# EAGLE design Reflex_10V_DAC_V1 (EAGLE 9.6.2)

## Sheet 1 of 3: Analog Circuits
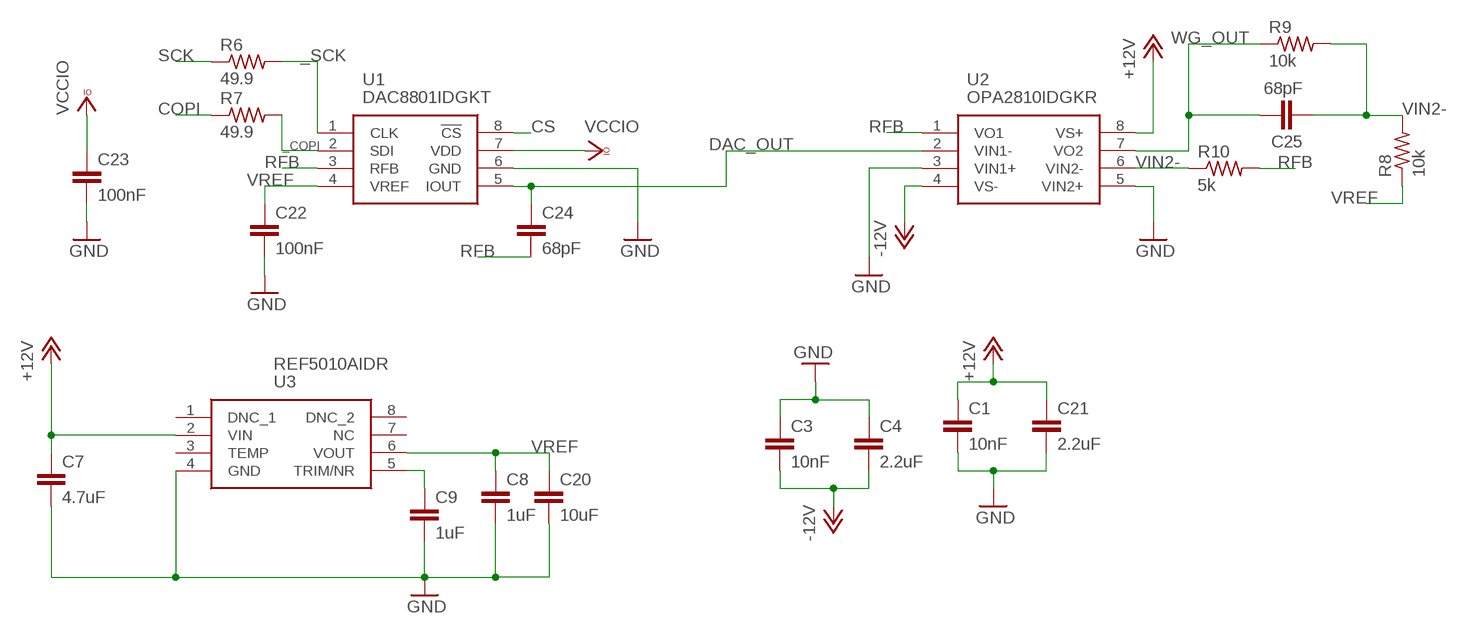
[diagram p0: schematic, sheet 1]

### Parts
C1  10nF  C-EUC0603  [C0603]
C3  10nF  C-EUC0603  [C0603]
C4  2.2uF  C-EUC0603  [C0603]
C7  4.7uF  C-EUC0603  [C0603]
C8  1uF  C-EUC0603  [C0603]
C9  1uF  C-EUC0603  [C0603]
C20  10uF  C-EUC0603  [C0603]
C21  2.2uF  C-EUC0603  [C0603]
C22  100nF  C-EUC0603  [C0603]
C23  100nF  C-EUC0603  [C0603]
C24  68pF  C-EUC0603  [C0603]
C25  68pF  C-EUC0603  [C0603]
R6  49.9  R-US_R0603  [R0603]
R7  49.9  R-US_R0603  [R0603]
R8  10k  R-US_R0603  [R0603]
R9  10k  R-US_R0603  [R0603]
R10  5k  R-US_R0603  [R0603]
U1  DAC8801IDGKT  [SOP65P490X110-8N]
U2  OPA2810IDGKR  [SOP65P490X110-8N]
U3  REF5010AIDR  [SOIC127P600X175-8N]

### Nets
+12V: C1.1 C7.1 C21.1 U2.8(VS+) U3.2(VIN) ; also sheet 2
-12V: C3.2 C4.2 U2.4(VS-) ; also sheet 2
_COPI: R7.2 U1.2(SDI)
_SCK: R6.2 U1.1(CLK)
COPI: R7.1 ; also sheet 3
CS: U1.8(!CS) ; also sheet 3
DAC_OUT: C24.1 U1.5(IOUT) U2.2(VIN1-)
GND: C1.2 C3.1 C4.1 C7.2 C8.2 C9.2 C20.2 C21.2 C22.2 C23.2 U1.6(GND) U2.3(VIN1+) U2.5(VIN2+) U3.4(GND) ; also sheet 2,3
N$8: C9.1 U3.5(TRIM/NR)
RFB: C24.2 R10.2 U1.3(RFB) U2.1(VO1)
SCK: R6.1 ; also sheet 3
VCCIO: C23.1 U1.7(VDD) ; also sheet 3
VIN2-: C25.2 R8.2 R9.2 R10.1 U2.6(VIN2-)
VREF: C8.1 C20.1 C22.1 R8.1 U1.4(VREF) U3.6(VOUT) ; also sheet 3
WG_OUT: C25.1 R9.1 U2.7(VO2) ; also sheet 3
Unconnected: U3.1(DNC_1) U3.3(TEMP) U3.7(NC) U3.8(DNC_2)

## Sheet 2 of 3: Power Circuits
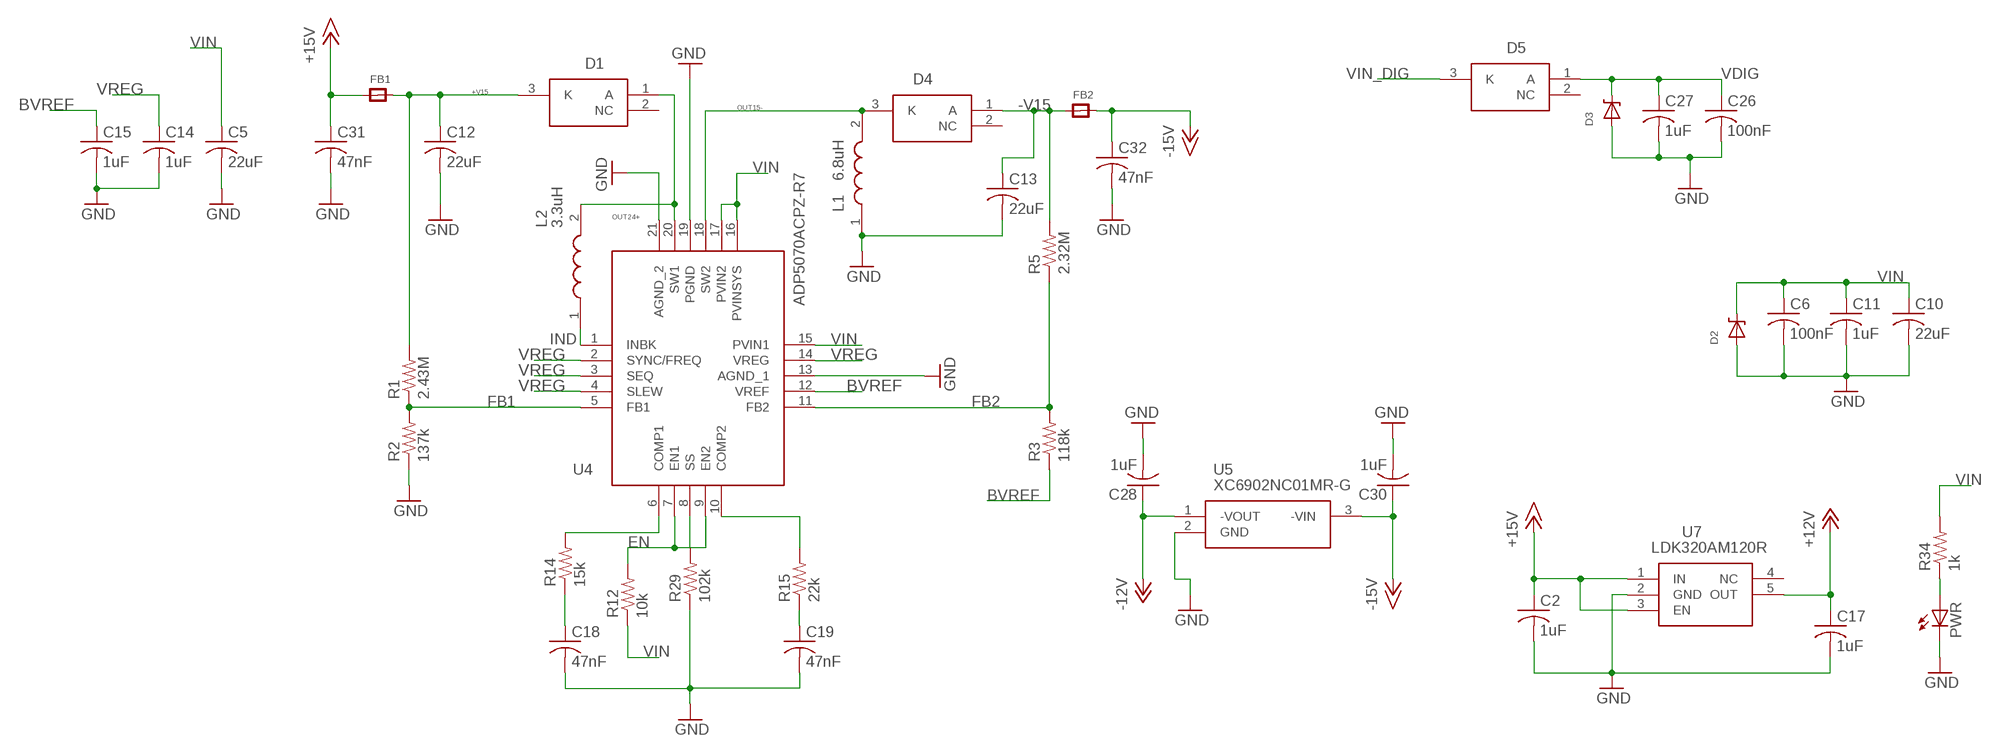
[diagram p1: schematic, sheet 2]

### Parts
C2  1uF  C-USC0603  [C0603]
C5  22uF  C-USC0603  [C0603]
C6  100nF  C-USC0603  [C0603]
C10  22uF  C-USC0603  [C0603]
C11  1uF  C-USC0603  [C0603]
C12  22uF  C-USC0805  [C0805]
C13  22uF  C-USC0805  [C0805]
C14  1uF  C-USC0603  [C0603]
C15  1uF  C-USC0603  [C0603]
C17  1uF  C-USC0603  [C0603]
C18  47nF  C-USC0603  [C0603]
C19  47nF  C-USC0603  [C0603]
C26  100nF  C-USC0603  [C0603]
C27  1uF  C-USC0603  [C0603]
C28  1uF  C-USC0603  [C0603]
C30  1uF  C-USC0603  [C0603]
C31  47nF  C-USC0603  [C0603]
C32  47nF  C-USC0603  [C0603]
D1  BAT54WFILMY  [SOT65P210X110-3N]
D2  DDZ5V6ASF  [DDZ5V6ASF]
D3  DDZ5V6ASF  [DDZ5V6ASF]
D4  BAT54WFILMY  [SOT65P210X110-3N]
D5  BAT54WFILMY  [SOT65P210X110-3N]
FB1  FERRITE  [0603]
FB2  FERRITE  [0603]
L1  6.8uH  MLZ2012M6R8HTD25  [INDC2012X105N]
L2  3.3uH  MLZ2012M4R7HT000  [INDC2012X145N]
PWR  LEDCHIPLED_0603  [CHIPLED_0603]
R1  2.43M  R-US_R0603  [R0603]
R2  137k  R-US_R0603  [R0603]
R3  118k  R-US_R0603  [R0603]
R5  2.32M  R-US_R0603  [R0603]
R12  10k  R-US_R0603  [R0603]
R14  15k  R-US_R0603  [R0603]
R15  22k  R-US_R0603  [R0603]
R29  102k  R-US_R0603  [R0603]
R34  1k  R-US_R0603  [R0603]
U4  ADP5070ACPZ-R7  [QFN50P400X400X80-21N]
U5  XC6902NC01MR-G  [SOT95P280X130-3N]
U7  LDK320AM120R  [SOT95P280X145-5N]

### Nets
+12V: C17.1 U7.5(OUT) ; also sheet 1
+15V: C2.1 C31.1 FB1.1 U7.1(IN) U7.3(EN)
+V15: C12.1 D1.3(K) FB1.2 R1.2
-12V: C28.1 U5.1(-VOUT) ; also sheet 1
-15V: C30.1 C32.1 FB2.2 U5.3(-VIN)
-V15: C13.1 D4.1(A) FB2.1 R5.2
BVREF: C15.1 R3.1 U4.12(VREF)
EN: R12.2 U4.7(EN1) U4.9(EN2) ; also sheet 3
FB1: R1.1 R2.2 U4.5(FB1)
FB2: R3.2 R5.1 U4.11(FB2)
GND: C2.2 C5.2 C6.2 C10.2 C11.2 C12.2 C13.2 C14.2 C15.2 C17.2 C18.2 C19.2 C26.2 C27.2 C28.2 C30.2 C31.2 C32.2 D2.P$1(A) D3.P$1(A) L1.1 PWR.C R2.1 R29.1 U4.13(AGND_1) U4.19(PGND) U4.21(AGND_2) U5.2(GND) U7.2(GND) ; also sheet 1,3
IND: L2.1 U4.1(INBK)
N$19: PWR.A R34.1
N$20: R29.2 U4.8(SS)
N$29: C18.1 R14.1
N$30: R14.2 U4.6(COMP1)
N$31: C19.1 R15.1
N$32: R15.2 U4.10(COMP2)
OUT15-: D4.3(K) L1.2 U4.18(SW2)
OUT24+: D1.1(A) L2.2 U4.20(SW1)
VDIG: C26.1 C27.1 D3.P$2(C) D5.1(A) ; also sheet 3
VIN: C5.1 C6.1 C10.1 C11.1 D2.P$2(C) R12.1 R34.2 U4.15(PVIN1) U4.16(PVINSYS) U4.17(PVIN2) ; also sheet 3
VIN_DIG: D5.3(K) ; also sheet 3
VREG: C14.1 U4.2(SYNC/FREQ) U4.3(SEQ) U4.4(SLEW) U4.14(VREG)
Unconnected: D1.2(NC) D4.2(NC) D5.2(NC) U7.4(NC)

## Sheet 3 of 3: Connectors and analog switch
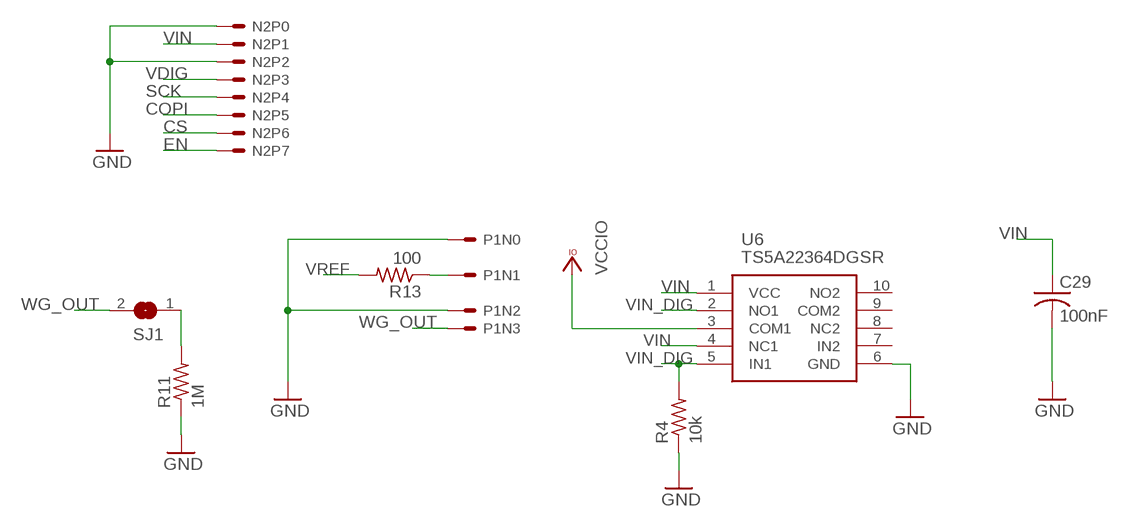
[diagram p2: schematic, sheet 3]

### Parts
C29  100nF  C-USC0603  [C0603]
N2  8PINHEADER  [8PINHEADER]
P1  4PINHEADER  [4PINHEADER]
R4  10k  R-US_R0603  [R0603]
R11  1M  R-US_R0603  [R0603]
R13  100  R-US_R0603  [R0603]
SJ1  SOLDERJUMPER  [SOLDERJUMPER_ARROW_NOPASTE]
U6  TS5A22364DGSR  [SOP50P490X110-10N]

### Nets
COPI: N2.P5 ; also sheet 1
CS: N2.P6 ; also sheet 1
EN: N2.P7 ; also sheet 2
GND: C29.2 N2.P0 N2.P2 P1.N0 P1.N2 R4.1 R11.1 U6.6(GND) ; also sheet 1,2
N$1: R11.2 SJ1.1
N$2: P1.N1 R13.1
SCK: N2.P4 ; also sheet 1
VCCIO: U6.3(COM1) ; also sheet 1
VDIG: N2.P3 ; also sheet 2
VIN: C29.1 N2.P1 U6.1(VCC) U6.4(NC1) ; also sheet 2
VIN_DIG: R4.2 U6.2(NO1) U6.5(IN1) ; also sheet 2
VREF: R13.2 ; also sheet 1
WG_OUT: P1.N3 SJ1.2 ; also sheet 1
Unconnected: U6.7(IN2) U6.8(NC2) U6.9(COM2) U6.10(NO2)

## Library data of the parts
C1 C3 C4 C7-C9 C20-C25 = rcl:C-EU: CAPACITOR, European symbol; SPICEPREFIX: C
C2 C5 C6 C10-C15 C17-C19 C26-C32 = rcl:C-US: CAPACITOR, American symbol; SPICEPREFIX: C
D1 D4 D5 = SamacSys_Parts:BAT54WFILMY: Automotive 40 V, 300 mA General purpose Small Signal Schottky Diode Source: Datasheet; DESCRIPTION: Automotive 40 V, 300 mA General purpose Small Signal Schottky Diode; HEIGHT: 1.1mm; MANUFACTURER_NAME: STMicroelectronics; MANUFACTURER_PART_NUMBER: BAT54WFILMY; MOUSER_PART_NUMBER: 511-BAT54WFILMY; MOUSER_PRICE-STOCK: https://www.mouser.co.uk/ProductDetail/STMicroelectronics/BAT54WFILMY?qs=aA7MvVR8Lz8Zb51n0tQT7w%3D%3D
D2 D3 = ForceTronics:DDZ5V6ASF: DDZ5V6ASF 5.42 Zener Diode
FB1 FB2 = microbuilder:FERRITE: Ferrite Bead
L1 = SamacSys_Parts:MLZ2012M6R8HTD25: The MLZ series include inductors for decoupling circuits that have top-class DC superimposition characteristics and low DC resistance. They are compatible with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; DESCRIPTION: The MLZ series include inductors for decoupling circuits that have top-class DC superimposition characteristics and low DC resistance. They are compatible with wide frequency band noise, from low to high frequency. H type products have a rated current that is equivalent to that of wound coils. W type products are the new standard type products that have both large current and low resistance. L type products have a resistance up to 60% lower than W type products. Operating temperature range: 55 to +125; HEIGHT: 1.05mm; MANUFACTURER_NAME: TDK; MANUFACTURER_PART_NUMBER: MLZ2012M6R8HTD25; MOUSER_PART_NUMBER: 810-MLZ2012M6R8HTD25; MOUSER_PRICE-STOCK: https://www.mouser.co.uk/ProductDetail/TDK/MLZ2012M6R8HTD25?qs=YdQ7Kj7W0bzS66dbWGL5AA%3D%3D
L2 = SamacSys_Parts:MLZ2012M4R7HT000: Inductor Power Shielded Multi-Layer 4.7uH 20% 2MHz Ferrite 0.4A 0.442Ohm DCR 0805 T/R; DESCRIPTION: Inductor Power Shielded Multi-Layer 4.7uH 20% 2MHz Ferrite 0.4A 0.442Ohm DCR 0805 T/R; HEIGHT: 1.45mm; MANUFACTURER_NAME: TDK; MANUFACTURER_PART_NUMBER: MLZ2012M4R7HT000; MOUSER_PART_NUMBER: 810-MLZ2012M4R7HT000; MOUSER_PRICE-STOCK: https://www.mouser.co.uk/ProductDetail/TDK/MLZ2012M4R7HT000?qs=%2FPzWLGNeQ%252BgQgMrI9kQ17A%3D%3D
N2 = ForceTronics:8PINHEADER: 8 pin header with 2.54mm spacing
P1 = ForceTronics:4PINHEADER
PWR = adafruit:LED: LED
R1-R15 R29 R34 = rcl:R-US_: RESISTOR, American symbol; SPICEPREFIX: R
SJ1 = microbuilder:SOLDERJUMPER: SMD Solder JUMPER; BOM: EXCLUDE
U1 = SamacSys_Parts:DAC8801IDGKT: 14-Bit, Single Channel, Serial Interface, Multiplying Digital-to-Analog Converter Source: Datasheet; DESCRIPTION: 14-Bit, Single Channel, Serial Interface, Multiplying Digital-to-Analog Converter; HEIGHT: 1.1mm; MANUFACTURER_NAME: Texas Instruments; MANUFACTURER_PART_NUMBER: DAC8801IDGKT; MOUSER_PART_NUMBER: 595-DAC8801IDGKT; MOUSER_PRICE-STOCK: https://www.mouser.co.uk/ProductDetail/Texas-Instruments/DAC8801IDGKT?qs=vul0MlC%2Fa1fY4dNbzQeDsA%3D%3D
U2 = SamacSys_Parts:OPA2810IDGKR: High Performance Low Cost Rail-to-Rail Input/Output HV FET Op Amps Source: Datasheet; DESCRIPTION: High Performance Low Cost Rail-to-Rail Input/Output HV FET Op Amps; HEIGHT: 1.1mm; MANUFACTURER_NAME: Texas Instruments; MANUFACTURER_PART_NUMBER: OPA2810IDGKR; MOUSER_PART_NUMBER: 595-OPA2810IDGKR; MOUSER_PRICE-STOCK: https://www.mouser.co.uk/ProductDetail/Texas-Instruments/OPA2810IDGKR?qs=YCa%2FAAYMW02J4dMmTpJlwg%3D%3D
U3 = SamacSys_Parts:REF5010AIDR: Low Noise, Very Low Drift, Precision Series Voltage Reference Source: Datasheet; DESCRIPTION: Low Noise, Very Low Drift, Precision Series Voltage Reference; HEIGHT: 1.75mm; MANUFACTURER_NAME: Texas Instruments; MANUFACTURER_PART_NUMBER: REF5010AIDR; MOUSER_PART_NUMBER: 595-REF5010AIDR; MOUSER_PRICE-STOCK: https://www.mouser.co.uk/ProductDetail/Texas-Instruments/REF5010AIDR?qs=XGzIaZb%2FFYJH5K17rhHGBw%3D%3D
U4 = SamacSys_Parts:ADP5070ACPZ-R7: ANALOG DEVICES - ADP5070ACPZ-R7 - DC/DC CONV, BOOST/INVERTING, LFCSP-20 Source: Datasheet; DESCRIPTION: ANALOG DEVICES - ADP5070ACPZ-R7 - DC/DC CONV, BOOST/INVERTING, LFCSP-20; HEIGHT: 0.8mm; MANUFACTURER_NAME: Analog Devices; MANUFACTURER_PART_NUMBER: ADP5070ACPZ-R7; MOUSER_PART_NUMBER: 584-ADP5070ACPZ-R7; MOUSER_PRICE-STOCK: https://www.mouser.co.uk/ProductDetail/Analog-Devices/ADP5070ACPZ-R7?qs=Ky1INM14uHq5PX2hKR%252Babw%3D%3D
U5 = SamacSys_Parts:XC6902NC01MR-G: Maximum Output Current : 200mA Input Voltage Range : -2.4 ~ -16V Output Voltage Range : -0.9 ~ -12V Accuracy : +/-1.5% for -2.0V ~ -12V +/-30mV (-0.9V ~ -1.95V) Temperature Stability : TYP. +/-50ppm/ Dropout Voltage : 400mVIOUT=100mA Low Power Consumption : 100uA Protection Circuits : Current Limit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; DESCRIPTION: Maximum Output Current : 200mA Input Voltage Range : -2.4 ~ -16V Output Voltage Range : -0.9 ~ -12V Accuracy : +/-1.5% for -2.0V ~ -12V +/-30mV (-0.9V ~ -1.95V) Temperature Stability : TYP. +/-50ppm/ Dropout Voltage : 400mVIOUT=100mA Low Power Consumption : 100uA Protection Circuits : Current Limit 350mA TYP. Foldback Thermal Shutdown (150) Output Capacitor : Ceramic Capacitor Compatible Operating Ambient Temperature : -40 ~ 85 Packages : SOT-23, SOT-89, USP-6C Environmentally Friendly : EU Ro; HEIGHT: 1.3mm; MANUFACTURER_NAME: Torex; MANUFACTURER_PART_NUMBER: XC6902NC01MR-G
U6 = SamacSys_Parts:TS5A22364DGSR: Analog Switch ICs 0.65-Ohm Dual SPDT Analog Switch Source: Datasheet; DESCRIPTION: Analog Switch ICs 0.65-Ohm Dual SPDT Analog Switch; HEIGHT: 1.1mm; MANUFACTURER_NAME: Texas Instruments; MANUFACTURER_PART_NUMBER: TS5A22364DGSR; MOUSER_PART_NUMBER: 595-TS5A22364DGSR; MOUSER_PRICE-STOCK: https://www.mouser.co.uk/ProductDetail/Texas-Instruments/TS5A22364DGSR?qs=9F2IyUQaA%2FhbjQmUI4VB%2FQ%3D%3D
U7 = SamacSys_Parts:LDK320AM120R: STMICROELECTRONICS - LDK320AM120R - LDO, FIXED, 12V, 0.2A, SOT-23-5 Source: Datasheet; DESCRIPTION: STMICROELECTRONICS - LDK320AM120R - LDO, FIXED, 12V, 0.2A, SOT-23-5; HEIGHT: 1.45mm; MANUFACTURER_NAME: STMicroelectronics; MANUFACTURER_PART_NUMBER: LDK320AM120R; MOUSER_PART_NUMBER: 511-LDK320AM120R; MOUSER_PRICE-STOCK: https://www.mouser.co.uk/ProductDetail/STMicroelectronics/LDK320AM120R?qs=wd5RIQLrsJgIHDY%252B%2Fbe1dQ%3D%3D

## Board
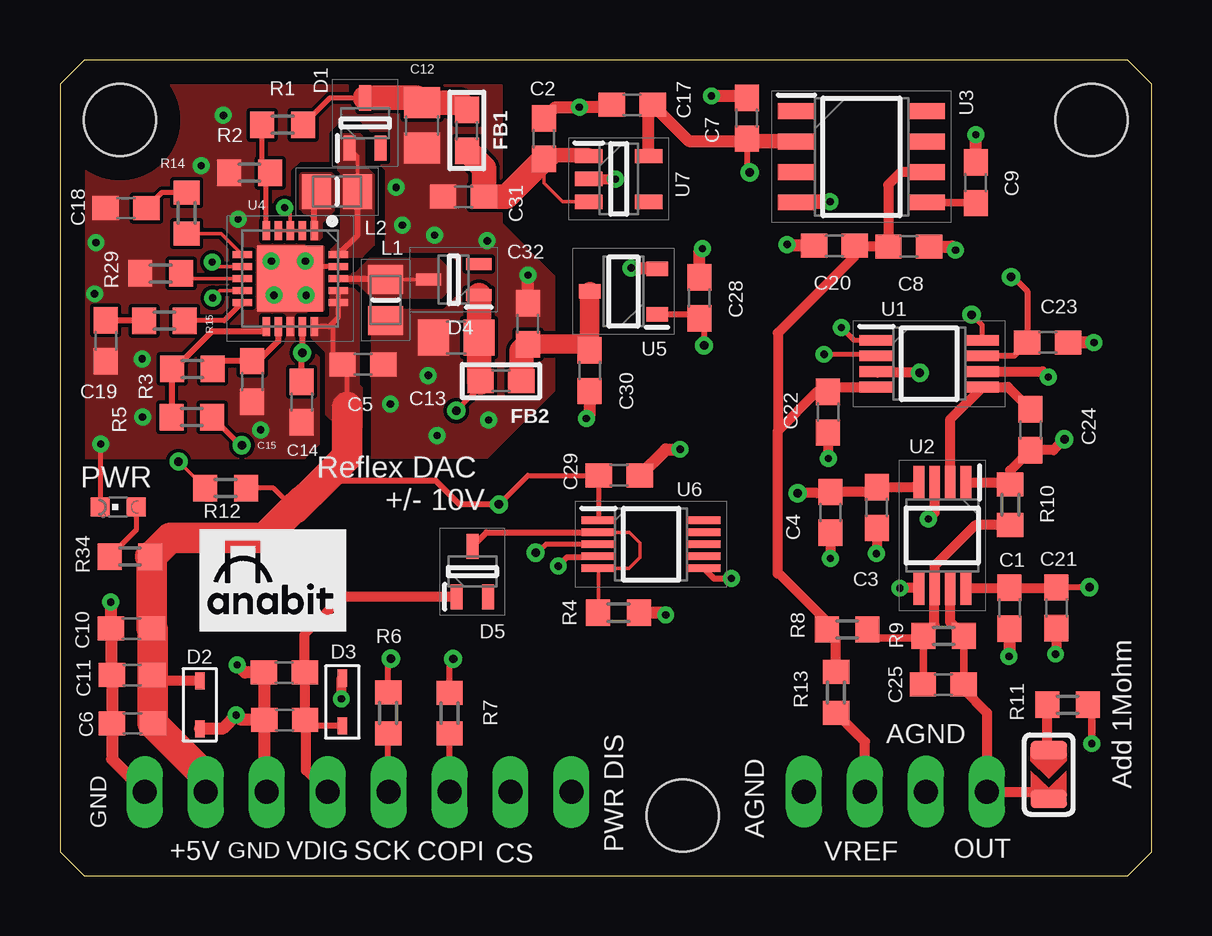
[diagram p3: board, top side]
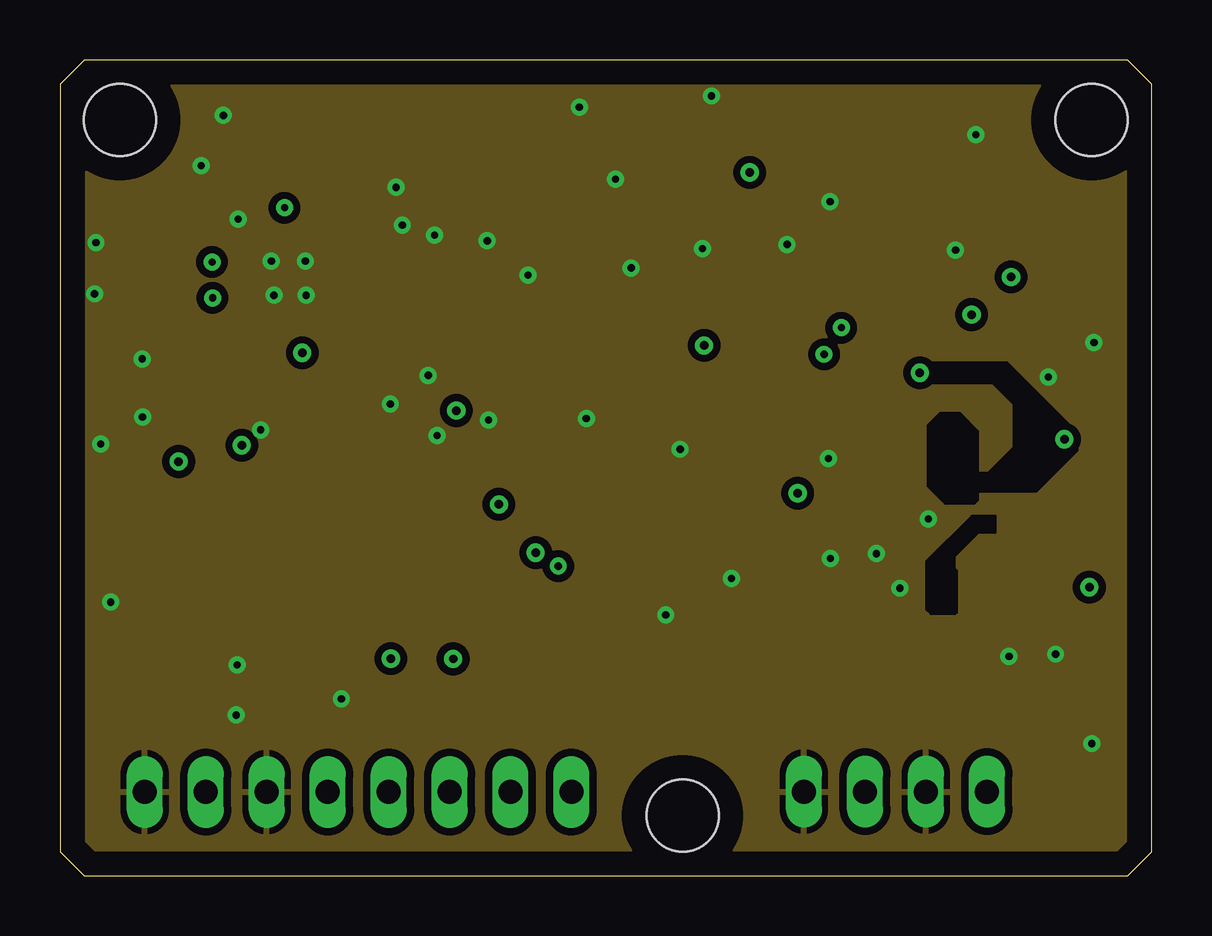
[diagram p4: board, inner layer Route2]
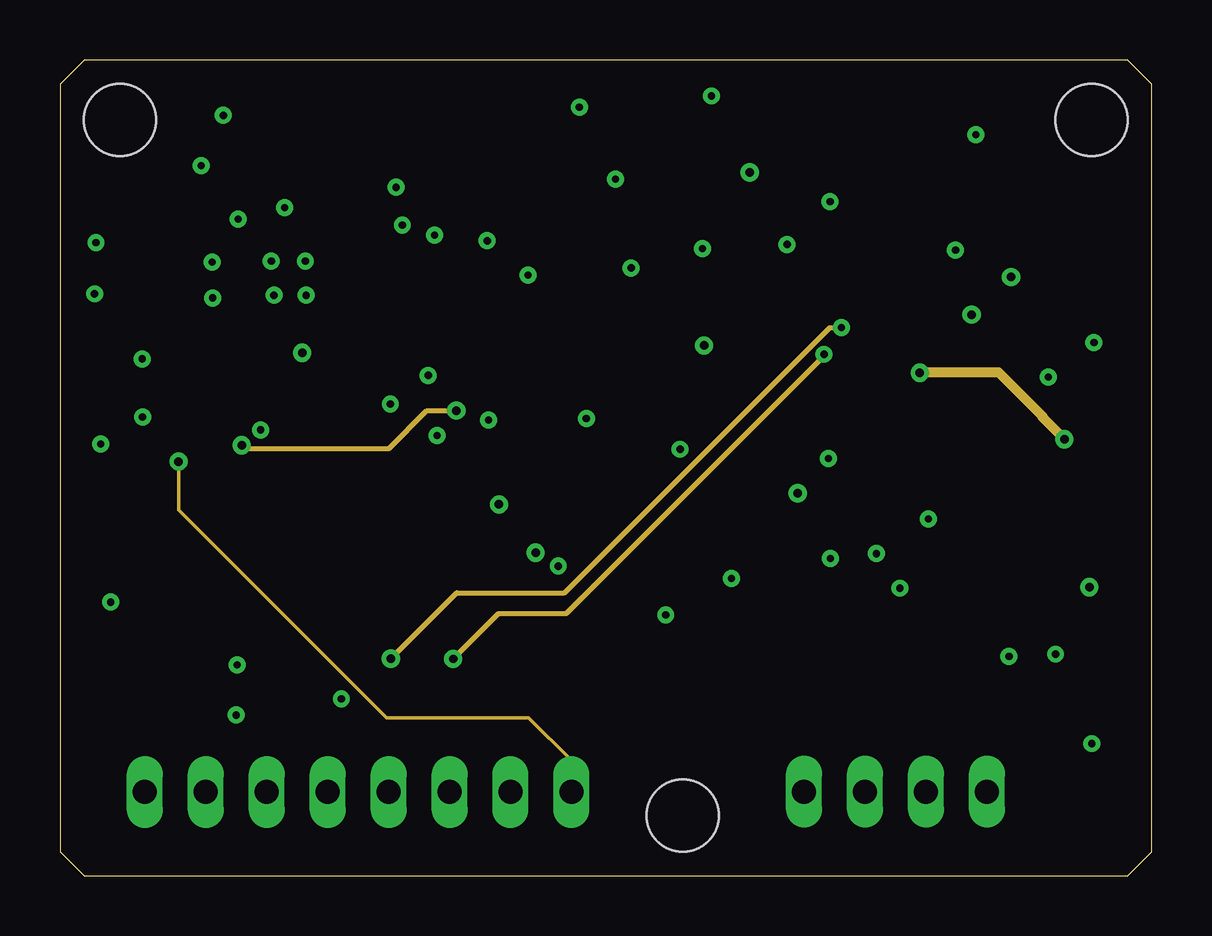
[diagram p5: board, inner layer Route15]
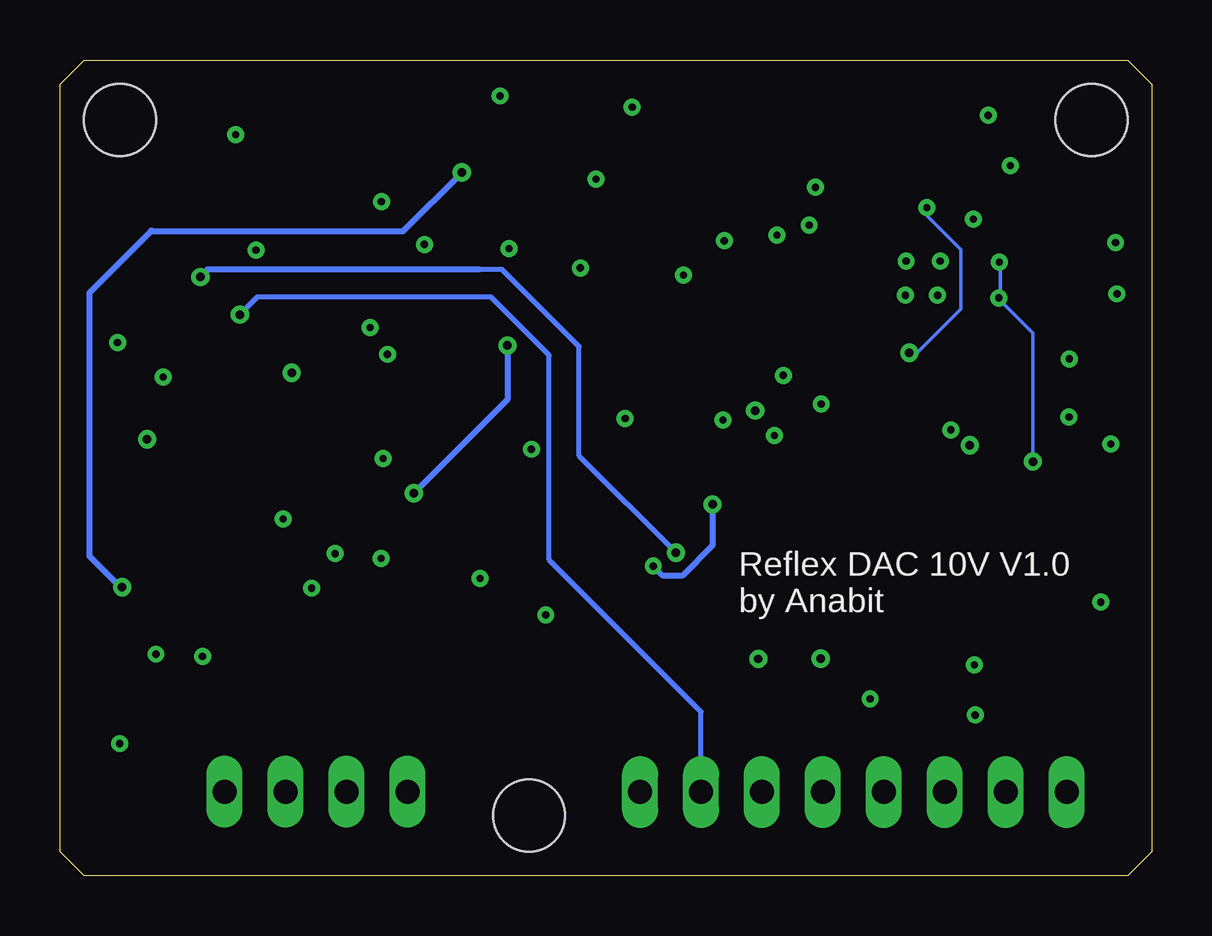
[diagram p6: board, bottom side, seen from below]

Size 45.5 x 34 mm. Coordinates in mm from the lower left corner, seen from the top.
Outline: 45.5,1 45.5,33 44.5,34 1,34 0,33 0,1 1,0 44.5,0 45.5,1
Copper layers (1+2*15+16): Top 0.035mm / dielectric 0.5mm / Route2 0.035mm / dielectric 0.6mm / Route15 0.035mm / dielectric 0.5mm / Bottom 0.035mm
Design rules "default *": minimum track width 6mil, minimum drill 0.3mm, track to track 6mil, track to pad 6mil, pad to pad 6mil, via to via 6mil, smd to smd 6mil, copper to edge 40mil, drill to drill 6mil, minimum pad ring 10mil, minimum via ring 8mil, stop-mask expansion 4mil, vias tented up to drill 0mil, thermal gap 10mil
Holes 3 mm at 2.5,31.5 25.95,2.5 43,31.5

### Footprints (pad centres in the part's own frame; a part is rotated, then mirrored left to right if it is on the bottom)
C0603 = smd 1.1 x 1: 1 -0.85,0; 2 0.85,0
C0805 = smd 1.3 x 1.5: 1 -0.95,0; 2 0.95,0
SOT65P210X110-3N = smd 1.05 x 0.5: 1 -1.05,0.65; 2 -1.05,-0.65; 3 1.05,0
DDZ5V6ASF = smd 0.71 x 0.41: P$1 0,0; P$2 1.99,0
0603 = smd 1.1 x 1: 1 -0.85,0; 2 0.85,0
INDC2012X105N = smd 1.2 x 1.45: 1 -0.85,0; 2 0.85,0
INDC2012X145N = smd 1.2 x 1.45: 1 -0.85,0; 2 0.85,0
8PINHEADER = drill 1 long: P0 1.27,-3.81; P1 3.81,-3.81; P2 6.35,-3.81; P3 8.89,-3.81; P4 11.43,-3.81; P5 13.97,-3.81; P6 16.51,-3.81; P7 19.05,-3.81
4PINHEADER = drill 1 long: N0 -3.81,0; N1 -1.27,0; N2 1.27,0; N3 3.81,0
CHIPLED_0603 = smd 0.8 x 0.8: A 0,-0.75; C 0,0.75
R0603 = smd 1 x 1.1: 1 -0.85,0; 2 0.85,0
SOLDERJUMPER_ARROW_NOPASTE = smd 0.762 x 1.524: 1 -1.016,0; 2 1.016,0
SOP65P490X110-8N = smd 1.4 x 0.45: 1 -2.2,0.975; 2 -2.2,0.325; 3 -2.2,-0.325; 4 -2.2,-0.975; 5 2.2,-0.975; 6 2.2,-0.325; 7 2.2,0.325; 8 2.2,0.975
SOIC127P600X175-8N = smd 1.528 x 0.65: 1 -2.711,1.905; 2 -2.711,0.635; 3 -2.711,-0.635; 4 -2.711,-1.905; 5 2.711,-1.905; 6 2.711,-0.635; 7 2.711,0.635; 8 2.711,1.905
QFN50P400X400X80-21N = smd 0.8 x 0.3: 1 -2,1; 2 -2,0.5; 3 -2,0; 4 -2,-0.5; 5 -2,-1; 11 2,-1; 12 2,-0.5; 13 2,0; 14 2,0.5; 15 2,1 | smd 0.3 x 0.8: 6 -1,-2; 7 -0.5,-2; 8 0,-2; 9 0.5,-2; 10 1,-2; 16 1,2; 17 0.5,2; 18 0,2; 19 -0.5,2; 20 -1,2 | smd 2.75 x 2.75: 21 0,0
SOT95P280X130-3N = smd 0.9 x 0.6: 1 -1.4,0.95; 2 -1.4,-0.95; 3 1.4,0
SOP50P490X110-10N = smd 1.4 x 0.3: 1 -2.2,1; 2 -2.2,0.5; 3 -2.2,0; 4 -2.2,-0.5; 5 -2.2,-1; 6 2.2,-1; 7 2.2,-0.5; 8 2.2,0; 9 2.2,0.5; 10 2.2,1
SOT95P280X145-5N = smd 1.15 x 0.6: 1 -1.25,0.95; 2 -1.25,0; 3 -1.25,-0.95; 4 1.25,-0.95; 5 1.25,0.95

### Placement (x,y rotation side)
C1  39.57,11.15 270 top
C2  20.18,30.72 90 top
C3  34.05,15.34 90 top
C4  32.12,15.14 90 top
C5  12.63,21.3 0 top
C6  3.02,6.35 180 top
C7  28.64,31.57 90 top
C8  35.38,26.22 0 top
C9  38.17,28.88 90 top
C10  2.98,10.3 180 top
C11  3.01,8.36 180 top
C12  15.09,31.27 270 top
C13  16.52,22.43 180 top
C14  10.07,19.74 270 top
C15  8.01,20.6 270 top
C17  23.85,32.14 180 top
C18  2.75,27.83 180 top
C19  1.91,22.29 270 top
C20  32.28,26.26 180 top
C21  41.54,11.16 270 top
C22  32.02,19.32 270 top
C23  41.17,22.22 0 top
C24  40.45,18.58 270 top
C25  36.82,7.97 180 top
C26  9.37,6.49 180 top
C27  9.35,8.46 180 top
C28  26.65,24.08 90 top
C29  23.31,16.68 0 top
C30  22.07,21.05 270 top
C31  16.82,28.3 180 top
C32  19.51,23 90 top
D1  12.72,31.37 90 top
D2  5.83,6.12 90 top
D3  11.77,8.23 270 top
D4  16.41,24.84 180 top
D5  17.19,12.67 90 top
FB1  16.96,31.06 90 top
FB2  18.38,20.61 0 top
L1  13.57,23.99 90 top
L2  11.55,28.51 0 top
N2  2.27,7.29 0 top
P1  34.83,3.5 0 top
PWR  2.43,15.36 90 top
R1  9.28,31.3 0 top
R2  7.9,29.3 0 top
R3  5.52,21.12 180 top
R4  23.28,10.96 180 top
R5  5.5,19.11 0 top
R6  13.68,6.78 90 top
R7  16.24,6.77 90 top
R8  32.81,10.26 0 top
R9  36.83,9.99 180 top
R10  39.61,15.46 90 top
R11  42,7.12 180 top
R12  6.91,16.15 180 top
R13  32.35,7.64 90 top
R14  5.28,27.62 270 top
R15  4.35,23.13 0 top
R29  4.2,25.1 0 top
R34  2.92,13.3 0 top
SJ1  41.21,4.21 270 top
U1  36.23,21.34 0 top
U2  36.78,14.18 270 top
U3  33.41,29.96 0 top
U4  9.6,24.88 270 top
U5  23.49,24.35 180 top
U6  24.64,13.81 0 top
U7  23.29,29.04 0 top

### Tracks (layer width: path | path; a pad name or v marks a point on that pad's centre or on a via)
+12V  (via drill 0.35)
  Top 0.254: v42.91,12.02 C21.1 | C7.1 28.64,29.38 28.73,29.29 v28.75,29.31
  Top 0.406: U2.8 37.77,12 C1.1 C21.1
  Top 0.508: U7.5 24.54,31.98 C17.1 26.22,30.62 28.74,30.62 28.84,30.62
  Top 0.61: 28.61,30.69 C7.1 28.74,30.62 | U3.2 30.36,30.59 30.33,30.62 28.84,30.62
  Bottom 0.254: 41.68,26.89 41.72,26.85 | 41.72,26.85 44.28,24.29 44.28,13.32 42.97,12.01 v42.92,12.01 v42.91,12.02 | v28.75,29.31 31.21,26.85 41.72,26.85
+15V
  Top 0.152: C2.1 20.18,28.86 20.95,28.09 U7.3
  Top 0.61: U7.1 22,30.03 20.64,30.03 20.48,29.87 C2.1
  Top 1.016: FB1.1 17.67,29.5 C31.1 18.61,28.3 C2.1
+V15
  Top 0.203: R1.2 11.25,32.42 D1.3
  Top 1.016: D1.3 14.89,32.42 C12.1 16.65,32.22 FB1.2
-12V  (via drill 0.35)
  Top 0.254: C4.2 31.82,15.69 31.57,15.94 | 33.85,15.99 C3.2 | U5.1 26.48,23.4 C28.1 26.84,23.04 v26.84,22.1 v26.85,22.1
  Top 0.406: 31.57,15.94 v30.75,15.94 | 33.85,15.99 C4.2 | C3.2 35.62,16.19 U2.4
  Bottom 0.254: v26.85,22.1 26.85,19.84 v30.75,15.94
-15V
  Top 0.813: C32.1 21.82,22.15 C30.1 22.07,24.33 U5.3
  Top 1.016: FB2.2 19.23,21.87 C32.1
-V15  (via drill 0.35)
  Top 0.152: D4.1
  Top 0.203: R5.2 7.53,17.93 v7.57,17.93 v7.58,17.94 | v16.52,19.38 17.53,20.39 17.53,20.55 FB2.1
  Top 1.016: D4.1 C13.1 17.47,20.61 17.53,20.55
  Route15 0.203: v7.58,17.94 7.71,17.81 13.72,17.81 15.29,19.38 v16.52,19.38
_COPI  (via drill 0.3, 0.35)
  Top 0.2: 31.87,21.71 33.92,21.71 33.88,21.66 U1.2
  Top 0.254: R7.2 16.24,8.9 v16.38,9.04 v16.39,9.03 | v31.85,21.73 31.87,21.71
  Route15 0.2: v16.39,9.03 18.28,10.92 21.11,10.92 31.89,21.7 v31.85,21.73
_SCK  (via drill 0.3, 0.35)
  Top 0.2: v32.57,22.84 33.09,22.32 U1.1
  Top 0.203: R6.2 13.68,7.84
  Top 0.254: R6.2 13.68,8.85 13.83,9 v13.79,9.04
  Route15 0.2: v13.79,9.04 16.54,11.79 21.04,11.79 32.09,22.84 v32.57,22.84
BVREF
  Top 0.254: U4.12 9.1,22.28 8.27,21.45 C15.1 6.7,21.45 R3.1
COPI
  Top 0.254: N2.P5 R7.1
CS  (via drill 0.35)
  Top 0.2: v38,23.38 38.43,22.95 U1.8
  Bottom 0.2: N2.P6 18.78,6.83 25.11,13.16 25.11,21.69 27.54,24.12 37.28,24.12 38,23.4 v38,23.38
DAC_OUT
  Top 0.406: U1.5 38.46,20.36 | 38.46,20.36 39.52,20.36 C24.1 | 38.46,20.36 37.1,19 U2.2
EN  (via drill 0.3, 0.35)
  Top 0.152: R12.2 v4.95,17.26 v4.95,17.25 | v6.36,24.08 6.66,24.38 U4.9 | v6.34,25.58 6.54,25.38 U4.7
  Route15 0.152: v4.95,17.25 4.95,15.24 13.61,6.58 19.54,6.58 21.32,4.8 N2.P7
  Bottom 0.152: v4.95,17.25 4.95,22.61 6.39,24.05 v6.36,24.08 6.3,24.14 6.3,25.54 v6.34,25.58
FB1
  Top 0.203: U4.5 8.6,29.15 R2.2 8.43,29.62 R1.1
FB2
  Top 0.254: U4.11 8.4,22.68 6.32,22.68 4.76,21.12 R3.2 4.65,21.1 R5.1
GNA
  cutout Route2 (no thermals): 39,15 38,15 36.1,13.1 36.1,11.1 36.3,10.9 37.3,10.9 37.4,11 37.4,12.7 37.3,12.8 37.3,13.3 38.3,14.3 39,14.3
GND  (via drill 0.3)
  Top 0.203: U4.19 10.46,25.38 v10.23,25.61 | v1.7,17.99 1.68,17.97 PWR.C
  Top 0.254: U6.6 27.27,12.38 v27.99,12.38
  Top 0.305: R11.1 43.01,6.96 v43.01,5.5
  Top 0.406: C4.1 v32.12,13.23 v32.11,13.22 | U1.6 40.97,21.02 v41.2,20.78 | C3.1 34.05,13.44 v34.03,13.42 | C22.2 v32.02,17.4 v32.03,17.39 | U2.3 36.45,15.12 v36.2,14.87 | C21.2 41.54,9.27 v41.5,9.23 | U2.5 v35.01,11.98 | U7.2 v23.15,29.04 v23.16,29.03 | v11.73,7.36 11.73,8.19 D3.P$1
  Top 0.508: v43.1,22.22 C23.2 | C1.2 v39.57,9.15 v39.56,9.14 | v2.12,11.4 v2.13,11.39 C10.2 2.16,10.27 C11.2 C6.2 2.17,4.85 N2.P0 | D2.P$1 6.78,6.12 v7.35,6.69 7.55,6.49 C26.2 | v7.38,8.78 7.7,8.46 C27.2 8.52,8.44 C26.2 | C26.2 8.52,3.58 N2.P2 | C2.2 20.64,32.03 v21.65,32.03 22.89,32.03 C17.2 | C7.2 28.56,32.5 v27.16,32.5 | C9.2 v38.17,30.87 v38.18,30.88 | C28.2 26.65,26.01 v26.78,26.14 | U5.2 23.84,25.3 v23.81,25.33 | C32.2 v19.51,25.03 | C30.2 22.07,19.18 v21.94,19.05 | C20.2 30.36,26.26 v30.31,26.31 | C8.2 37.18,26.22 v37.33,26.07 | C29.2 25.25,17.77 v25.85,17.77 | R4.1 25.15,10.96 v25.25,10.86
  Top 0.61: U3.4 30.73,28.09 v32.1,28.09
  other vias: 8.37,18.58 15.35,20.85 8.81,25.62 8.92,24.19 10.26,24.19 13.77,19.66 14.01,28.69 14.27,27.11 5.88,29.59 3.43,21.54 3.44,19.11 1.44,24.25 1.5,26.38 7.43,27.37 6.81,31.69 15.62,26.7 15.72,18.34 17.86,18.99 17.81,26.46
  pour Route2 (isolate 0.305): -1,35 47,35 48.5,33.5 48.5,0.5 45.5,-2.5 0.5,-2.5 -1.5,-0.5 -1.5,34.5
  cutout Route2: 36.18,16.22 36.18,18.78 36.7,19.3 37.5,19.3 38.26,18.54 38.26,15.64 38.12,15.5 36.9,15.5
  cutout Route2: 36.4,21.4 39.46,21.4 42.4,18.46 42.4,17.7 40.7,16 38.4,16 38.2,16.2 38.2,16.8 38.7,16.8 39.77,17.87 39.77,19.64 38.89,20.52 36.4,20.52
  pour Top (no thermals): -1.2,17.4 10.2,17.4 10.8,18 10.8,21.6 10.2,22.2 10.2,23.4 10.4,23.6 11,23.6 11,26.2 10.2,26.2 10.2,27 9.6,27.6 9.6,29.4 10,29.8 11.2,29.8 11.2,31 12,31.8 12,34.4 -0.8,34.4 -0.8,17.8
  pour Top (no thermals): 13,17.4 13,23.6 16,23.6 16.6,24.2 16.6,25.6 16.2,26 13.6,26 13.6,29.4 13.4,29.6 13.4,30.6 12.4,31.6 11.6,31.6 11.6,35.6 18.4,35.6 18.4,27.2 20.6,25 20.6,20.2 17.8,17.4
IND
  Top 0.254: U4.1 10.6,28.41 L2.1
  pour Top (no thermals): 10.5,26.5 10.5,27.4 10.3,27.6 10.2,27.6 10,27.8 10,29.2 10.1,29.3 11.3,29.3 11.4,29.2 11.4,27.7 10.9,27.2 10.9,26.6 10.8,26.5
N$1
  Top 0.406: SJ1.1 41.15,5.29 R11.2
N$2
  Top 0.406: P1.N1 33.56,5.58 R13.1
N$8
  Top 0.305: U3.5 38.15,28.05 C9.1
N$19
  Top 0.203: PWR.A 3.18,14.41 R34.1
N$20
  Top 0.152: U4.8 5.27,24.88 R29.2
N$29
  Top 0.203: R14.1 4.24,28.47 C18.1
N$30
  Top 0.152: U4.6 6.71,26.77 R14.2
N$31
  Top 0.254: R15.1 C19.1
N$32
  Top 0.203: U4.10 6.85,23.13 R15.2
OUT15-
  Top 0.152: L1.2 D4.3
  Top 0.254: U4.18 13.53,24.88 L1.2
  pour Top (no thermals): 12.1,25 11.3,25 11.3,24.8 12,24.8 12.1,24.7 12.4,24.7 13,24.1 15.9,24.1 16.2,24.4 16.2,25.3 15.8,25.7 12.9,25.7 12.3,25.1 12.2,25.1
OUT24+
  Top 0.152: D1.1 12.4,29.99 L2.2
  Top 0.254: U4.20 12.4,26.68 L2.2
  pour Top (no thermals): 12.5,30.9 11.8,30.9 11.6,30.7 11.6,29.4 11.7,29.3 11.7,26.5 11.3,26.1 11.3,25.8 12.6,25.8 13.1,26.3 13.1,29.2 12.7,29.6 12.7,30.7
RFB  (via drill 0.35)
  Top 0.305: R10.2 39.45,16.31 39.37,16.39 | 34.09,20.96 U1.3
  Top 0.406: v35.84,20.96 34.09,20.96 | v41.87,18.19 41.41,17.73 C24.2 39.61,16.89 R10.2 39.54,16.38 U2.1
  Route15 0.406: v35.84,20.96 v35.84,20.97 39.13,20.97 40.96,19.14 40.96,19.1 v41.87,18.19
SCK
  Top 0.254: N2.P4 13.68,3.5 R6.1
VCCIO  (via drill 0.35)
  Top 0.203: U6.3 20.25,13.81 19.86,13.43 v19.83,13.46
  Top 0.254: v39.65,24.95 39.73,24.95 40.32,24.37 C23.1 39.77,21.66 U1.7 | 22.41,13.78 U6.3
  Bottom 0.203: v19.83,13.46 23.86,17.49 23.86,22.06 27.07,25.27 28.15,25.27
  Bottom 0.254: v39.65,24.95 39.65,24.98 39.35,25.27 28.15,25.27 28.03,25.27
VDIG
  Top 0.254: D3.P$2 10.47,6.24 10.26,6.45 C26.1
  Top 0.406: N2.P3 10.26,4.38 10.26,6.45 | C26.1 10.22,8.44 C27.1 10.2,10.07 11.75,11.62 D5.1
VIN  (via drill 0.3, 0.35)
  Top 0.2: U4.17 U4.16 11.6,23.27 11.37,23.04 | U4.15 11.21,22.88 11.37,23.04 | 11.37,23.04 11.37,21.71 C5.1
  Top 0.203: 11.97,19.54 11.97,21.11 C5.1 | v18.3,15.47 19.5,16.68 C29.1 22.44,16.66 U6.1 | 9.75,15.3 8.9,16.15 R12.1
  Top 0.254: U6.4 22.41,13.28 21.15,13.28 v20.77,12.9 | 10.98,16.48 15.65,16.48 16.66,15.47 v18.3,15.47
  Top 0.406: D2.P$2 3.87,8.11
  Top 0.61: C10.1 3.77,10.36
  Top 0.813: C11.1 | 3.86,10.27 C10.1 4.08,10.05 | 6.08,4.14 N2.P1
  Top 1.27: C11.1 3.87,8.11 C6.1 6.08,4.14 | C11.1 3.86,10.27 | C10.1 3.83,13.24 R34.2 3.83,13.3 4.6,14.07 8.52,14.07 9.75,15.3 | 9.75,15.3 10.05,15.6 | 11.97,19.54 11.97,17.46 10.98,16.48 9.81,15.3 9.75,15.3
  Bottom 0.254: v18.3,15.47 18.3,13.77 19.54,12.52 20.39,12.52 v20.77,12.9
  pour Top (no thermals): 10.47,23.24 10.47,22.44 11.07,21.84 11.07,19.24 11.67,18.64 12.59,18.64 12.59,20.32 12.47,20.44 12.47,24.24 12.27,24.44 11.27,24.44 11.27,23.34 11.17,23.24
VIN2-
  Top 0.305: R9.2 35.98,9.9 | 35.98,9.9 C25.2 | R8.2 34.02,9.9 35.98,9.9
  Top 0.406: R10.1 38.16,14.61 36.45,12.9 U2.6 36.45,10.46 R9.2
VIN_DIG
  Top 0.152: R4.2 22.44,11.32 U6.5 23.71,12.81 24.17,13.27 24.17,13.87 23.73,14.31 U6.2
  Top 0.254: D5.3 17.78,14.31 U6.2
VREF
  Top 0.203: R8.1 31.96,10.59 | C22.1 31.74,20.17
  Top 0.254: 31.76,20.17 C22.1 32.22,20.36
  Top 0.305: 29.95,12.61 29.92,12.58 | 31.56,20.17 C22.1 | 33.17,26.22 C20.1
  Top 0.406: R13.2 32.35,9.87 R8.1 | 32.22,20.36 U1.4 | 29.95,12.61 31.96,10.59 | 29.92,12.58 29.92,18.53 | 29.92,18.53 31.56,20.17 | U3.6 35.05,29.32 34.53,28.8 C8.1 33.17,26.22 | C20.1 33.13,25.83 29.92,22.62 29.92,18.53
VREG  (via drill 0.3, 0.35)
  Top 0.152: v9.36,27.84 9.6,27.6 U4.3 | U4.3 U4.4 | U4.3 U4.2
  Top 0.254: U4.14 v10.1,21.79 10.1,21.68 10.07,21.65 C14.1
  Bottom 0.152: v10.1,21.79 9.78,21.79 7.95,23.62 7.95,26.1 9.36,27.51 v9.36,27.84
WG_OUT
  Top 0.305: R9.1 C25.1
  Top 0.406: C25.1 37.67,7.76 38.64,6.79 P1.N3 40.9,3.5 SJ1.2 | R9.1 37.1,10.56 U2.7

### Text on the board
tNames: Reflex DAC / +/- 10V | AGND | AGND | GND | Add 1Mohm | +5V | GND | VDIG | SCK | COPI | CS | PWR DIS | VREF | OUT
bNames: Reflex DAC 10V V1.0 / by Anabit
